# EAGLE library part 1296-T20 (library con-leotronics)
1.27mm SINGLE ROW FEMALE SOCKET Source: http://www.leotronics.co.uk/Conexcon/Data%20Sheets/sec.%20A/1296ing.pdf
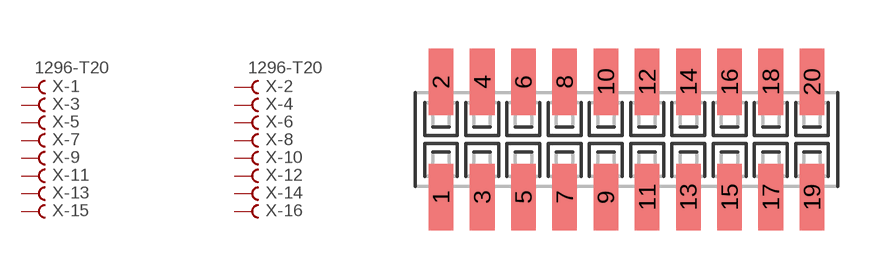
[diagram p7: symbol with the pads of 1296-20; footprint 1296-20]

Designator prefix X; gates -1=FVAL -2=FVAL -3=F -4=F -5=F -6=F -7=F -8=F -9=F -10=F -11=F -12=F -13=F -14=F -15=F -16=F -17=F -18=F -19=F -20=F

## 1296-T20 (OC_FARNELL: unknown; OC_NEWARK: unknown)  [1296-20]
1  -1:B  pas
2  -2:B  pas
3  -3:B  pas
4  -4:B  pas
5  -5:B  pas
6  -6:B  pas
7  -7:B  pas
8  -8:B  pas
9  -9:B  pas
10  -10:B  pas
11  -11:B  pas
12  -12:B  pas
13  -13:B  pas
14  -14:B  pas
15  -15:B  pas
16  -16:B  pas
17  -17:B  pas
18  -18:B  pas
19  -19:B  pas
20  -20:B  pas

## Footprint 1296-20 (pad centres in mm)
1.27mm SINGLE ROW FEMALE SOCKET Source: http://www.leotronics.co.uk/Conexcon/Data%20Sheets/sec.%20A/1296ing.pdf
smd 0.76 x 2.05: 1 -5.715,-1.78; 2 -5.715,1.78; 3 -4.445,-1.78; 4 -4.445,1.78; 5 -3.175,-1.78; 6 -3.175,1.78; 7 -1.905,-1.78; 8 -1.905,1.78; 9 -0.635,-1.78; 10 -0.635,1.78; 11 0.635,-1.78; 12 0.635,1.78; 13 1.905,-1.78; 14 1.905,1.78; 15 3.175,-1.78; 16 3.175,1.78; 17 4.445,-1.78; 18 4.445,1.78; 19 5.715,-1.78; 20 5.715,1.78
